
DATA_BLOCK DB22
TITLE =   <interner Baustein-Titel/ Internal block title>


AUTHOR:   Andy     //  max. 8 Zeichen / max. 8 characters
FAMILY:   plant1   //  max. 8 Zeichen / max. 8 characters
NAME:     db_mot1  //  max. 8 Zeichen / max. 8 characters
VERSION:  01.01    //  max. 15.15


STRUCT
a       { S7_m_c := 'true' }   :       bool    :=             1;       //1
b       { S7_m_c := 'true' }   :       byte    :=      b#16#1  ;       //2
c       { S7_m_c := 'true' }   :       word    :=      w#16#2  ;       //3
d       { S7_m_c := 'true' }   :       int     :=      3       ;       //4
e       { S7_m_c := 'true' }   :       dint    :=      l#4     ;       //5
f       { S7_m_c := 'true' }   :       real    :=      5.00    ;       //6
g       { S7_m_c := 'true' }   :       real    :=      6.00    ;       //7
END_STRUCT;

BEGIN
 END_DATA_BLOCK

